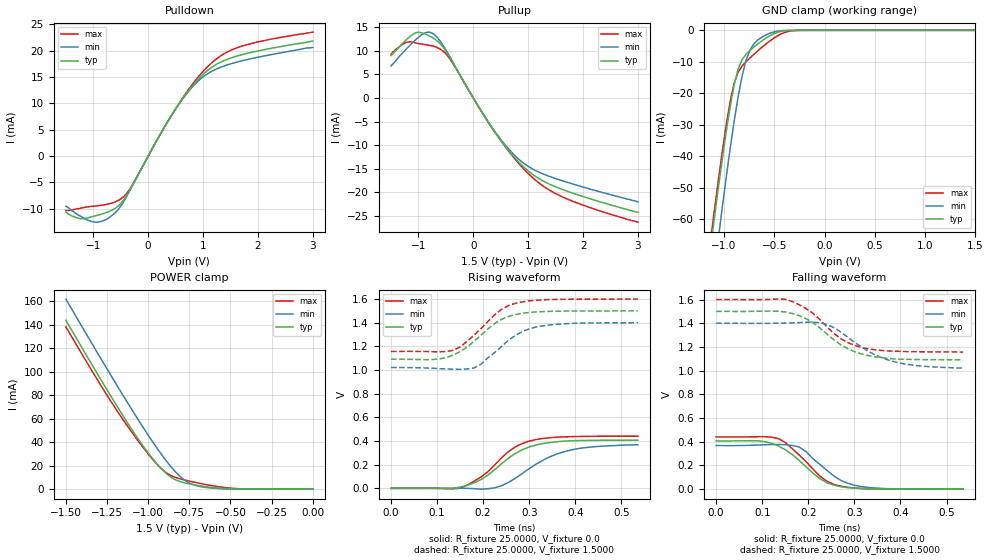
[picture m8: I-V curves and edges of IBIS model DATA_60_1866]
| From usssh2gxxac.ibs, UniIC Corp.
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|   Model DATA_60_1866
[Model]  DATA_60_1866
Model_type I/O
Polarity   Non-Inverting
Enable   Active-High
Vinl =   0.61500000V
Vinh =   0.88500000V
Vmeas =   0.750000000V
Rref =   25.00000000
Vref =   0.75000000V
C_comp   1.6160pF   1.5990pF   1.6430pF
[Temperature Range]   25.0000   95.0000   0.0
[Voltage Range]   1.5000V   1.4000V   1.6000V
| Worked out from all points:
|   slope of the pulldown table from 0 to 0.225 V, typ, clamps not added: 53.4 ohm
|   slope of the pullup table from 0 to 0.225 V, typ, clamps not added: 52.6 ohm
|   GND clamp passes 1 mA (typ) near -0.50 V on its own axis
|   POWER clamp passes 1 mA (typ) near -0.58 V on its own axis
|   rising waveform, R_fixture 25.0000, V_fixture 0.0: 20-80 % time 86.5ps typ, 98.3ps min, 79ps max; typ from 0 V to 0.407 V
|   rising waveform, R_fixture 25.0000, V_fixture 1.5000: 20-80 % time 78.8ps typ, 76.1ps min, 73.4ps max; typ from 1.09 V to 1.5 V
|   falling waveform, R_fixture 25.0000, V_fixture 0.0: 20-80 % time 75.8ps typ, 70.4ps min, 70.8ps max; typ from 0.407 V to 0 V
|   falling waveform, R_fixture 25.0000, V_fixture 1.5000: 20-80 % time 88.4ps typ, 97.1ps min, 81.8ps max; typ from 1.5 V to 1.09 V
[Pulldown]
|Voltage   I(typ)   I(min)   I(max)
-1.5V     -10.6mA    -9.5mA     -10.3mA
-1.25V    -11.86mA   -11.3mA    -9.93mA
-1V       -11.42mA   -12.48mA   -9.5mA
-800mV    -10.84mA   -12.17mA   -9.25mA
-600mV    -9.882mA   -10.74mA   -8.682mA
-350mV    -6.704mA   -6.838mA   -6.505mA
200mV     3.763mA    3.796mA    3.76mA
550mV     9.696mA    9.684mA    9.781mA
850mV     13.86mA    13.59mA    14.19mA
1.15V     16.76mA    16.02mA    17.61mA
1.75V     19.33mA    18.16mA    20.97mA
3V        21.8mA     20.6mA     23.5mA
[Pullup]
|Voltage   I(typ)   I(min)   I(max)
-1.5V     9mA        6.8mA      9.3mA
-1.25V    12.03mA    10mA       11.63mA
-1.05V    13.82mA    12.36mA    11.68mA
-900mV    13.65mA    13.69mA    11.34mA
-750mV    12.84mA    13.77mA    11.04mA
-600mV    11.47mA    12.01mA    10.35mA
-450mV    9.041mA    9.198mA    8.665mA
300mV     -5.62mA    -5.548mA   -5.6mA
850mV     -13.84mA   -13.18mA   -14.16mA
1.2V      -17.1mA    -15.73mA   -18.03mA
1.55V     -19.04mA   -17.25mA   -20.54mA
3V        -24.2mA    -22mA      -26.3mA
[GND_clamp]
|Voltage   I(typ)   I(min)   I(max)
-1.5V     -169mA     -189.1mA   -163.8mA
-1.14V    -70.71mA   -88.3mA    -68.32mA
-1.1V     -60.74mA   -77.66mA   -58.33mA
-1.06V    -51.03mA   -67.22mA   -48.61mA
-1.02V    -41.65mA   -57.06mA   -39.27mA
-940mV    -24.55mA   -37.9mA    -22.88mA
-860mV    -12.39mA   -21.26mA   -13.32mA
-780mV    -7.577mA   -9.433mA   -9.942mA
-740mV    -6.329mA   -6.125mA   -8.71mA
-620mV    -3.273mA   -2.113mA   -5.305mA
-300mV    -11.81uA   -4.878uA   -91.71uA
1.5V      4.577nA    23.6nA     33.33nA
[POWER_clamp]
|Voltage   I(typ)   I(min)   I(max)
-1.5V     143.7mA    161.7mA    138.1mA
-1.22V    77.56mA    95.29mA    73.32mA
-1.12V    55.19mA    72.34mA    52.54mA
-1.02V    34.59mA    50.23mA    33.56mA
-960mV    23.77mA    37.63mA    23.28mA
-900mV    14.66mA    25.9mA     15mA
-840mV    8.415mA    15.63mA    10.28mA
-780mV    5.408mA    7.848mA    7.861mA
-700mV    3.206mA    2.693mA    5.332mA
-600mV    1.29mA     794.5uA    2.681mA
-420mV    69.47uA    44.47uA    238.7uA
0V        4.577nA    6.249nA    39.08nA
[Ramp]
| variable   typ   min   max
dV/dt_r  0.2442/86.5366p   0.2207/98.3857p   0.2647/78.9981p
dV/dt_f  0.2448/88.3671p   0.2280/97.6364p   0.2658/81.8205p
R_load = 25.0000
[Rising Waveform]
R_fixture= 25.0000
V_fixture= 0.0
V_fixture_min= 0.0
V_fixture_max= 0.0
|time   V(typ)   V(min)   V(max)
0s        0V         0V         0V
120ps     -2.381mV   528.8uV    -1.509mV
150ps     10.65mV    548.9uV    1.139mV
195ps     73.7mV     -6.902mV   95.42mV
240ps     208.5mV    22.31mV    258.4mV
270ps     295.1mV    85.55mV    351.1mV
315ps     367.2mV    204.9mV    412.7mV
360ps     393.6mV    290.1mV    432.3mV
405ps     403.9mV    335.2mV    438.4mV
536ps     407mV      367.8mV    441.2mV
[Rising Waveform]
R_fixture= 25.0000
V_fixture= 1.5000
V_fixture_min= 1.4000
V_fixture_max= 1.6000
|time   V(typ)   V(min)   V(max)
0s        1.092V     1.021V     1.157V
90.91ps   1.089V     1.015V     1.155V
135ps     1.126V     1.007V     1.167V
180ps     1.242V     1.017V     1.294V
195ps     1.294V     1.048V     1.349V
240ps     1.429V     1.2V       1.513V
270ps     1.469V     1.293V     1.564V
300ps     1.487V     1.348V     1.585V
345ps     1.496V     1.382V     1.596V
536ps     1.5V       1.4V       1.6V
[Falling Waveform]
R_fixture= 25.0000
V_fixture= 0.0
V_fixture_min= 0.0
V_fixture_max= 0.0
|time   V(typ)   V(min)   V(max)
0s        407mV      367.9mV    441.2mV
90.91ps   407.1mV    372.3mV    442.5mV
135ps     365mV      377.3mV    426.7mV
180ps     242.9mV    355.8mV    288.3mV
225ps     89.18mV    210mV      110.1mV
240ps     55.03mV    159.7mV    67.61mV
270ps     21.56mV    75.55mV    25.62mV
300ps     8.296mV    33.1mV     9.851mV
345ps     2.071mV    9.369mV    2.344mV
536ps     0V         0V         0V
[Falling Waveform]
R_fixture= 25.0000
V_fixture= 1.5000
V_fixture_min= 1.4000
V_fixture_max= 1.6000
|time   V(typ)   V(min)   V(max)
0s        1.5V       1.4V       1.6V
150ps     1.495V     1.401V     1.602V
195ps     1.439V     1.409V     1.524V
225ps     1.361V     1.404V     1.431V
240ps     1.31V      1.39V      1.371V
270ps     1.22V      1.328V     1.271V
315ps     1.141V     1.2V       1.196V
360ps     1.11V      1.108V     1.17V
405ps     1.096V     1.059V     1.162V
536ps     1.092V     1.021V     1.157V
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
